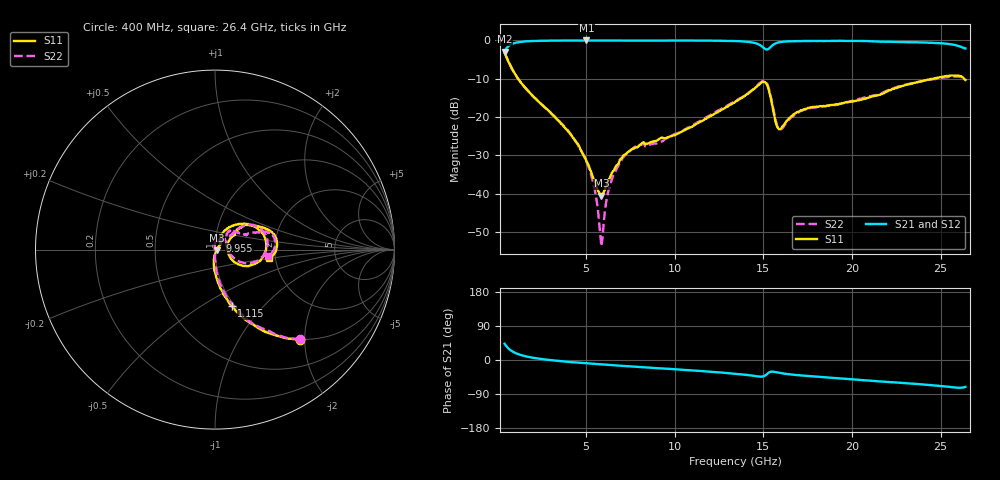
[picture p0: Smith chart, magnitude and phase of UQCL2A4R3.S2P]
! AVX Corporation
! Date:  10/27/06
! Part No:  UQCL2A4R3
! Description:  Ultra Low ESR Microwave capacitors
! Mounting Orientation:  Horizontal
# GHZ S DB R 50
! Freq  |S11|  S11 Ph  |S21|  S21 Ph  |S12|  S12 Ph  |S22|  S22 Ph
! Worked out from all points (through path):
!   401 points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, 400 MHz to 26.4 GHz, reference 50 ohm
!   highest |S21| = -0.04 dB at 5.015 GHz (marker M1); lowest = -2.9 dB at 400 MHz (marker M2)
!   group delay of S21, straight-line fit = 8.74 ps
!   lowest |S11| = -40.5 dB at 5.86 GHz (marker M3), VSWR 1.02, Z = 50.9 - j0.397 ohm
!   |S11| at or under -10 dB: 1.158 GHz to 24.58 GHz (23.42 GHz wide, 182 % of centre); 26.32633 GHz to end of sweep
!   |S22| runs from -53.7 to -3.2 dB; largest |S21 - S12| = 0.0084
!   S11 on the Smith chart (normalised r, x): 400 MHz: 0.99, -1.89; 1.115 GHz: 0.97, -0.68; 9.955 GHz: 1.05, +0.11; 26.4 GHz: 1.84, -0.20
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0.4  -3.23 -46.7  -2.93 42.7  -2.97 42.7  -3.23 -46.5
1.115  -9.72 -73.4  -0.54 16.4  -0.57 16.3  -9.69 -72.4
3.91  -23.34 -95.5  -0.06 -4.6  -0.04 -4.6  -23.16 -88.2
4.755  -29.09 -95.0  -0.05 -7.8  -0.04 -7.9  -29.14 -89.2
5.015  -31.53 -90.7  -0.04 -8.8  -0.03 -8.8  -31.63 -90.0
5.47  -36.68 -72.0  -0.04 -10.4  -0.03 -10.4  -38.60 -95.9
5.86  -40.54 -24.5  -0.04 -11.7  -0.04 -11.7  -53.72 -175.2
6.315  -36.07 23.3  -0.06 -13.2  -0.05 -13.1  -38.18 97.6
7.03  -30.59 40.2  -0.06 -15.4  -0.03 -15.5  -30.96 94.5
7.81  -27.96 44.7  -0.06 -17.8  -0.04 -18.0  -27.74 85.9
9.11  -25.76 56.9  -0.08 -21.8  -0.08 -22.0  -26.60 71.2
9.955  -24.77 61.1  -0.07 -24.3  -0.05 -24.4  -24.55 57.6
13.4  -16.13 55.5  -0.21 -36.1  -0.21 -36.1  -15.86 41.9
14.57  -12.27 33.8  -0.77 -42.7  -0.79 -42.5  -12.18 34.1
15.09  -10.92 0.2  -2.22 -41.2  -2.24 -41.2  -10.62 5.1
15.415  -14.98 -30.5  -1.73 -31.1  -1.75 -31.1  -14.55 -23.9
15.74  -22.09 -18.4  -0.71 -32.4  -0.73 -32.3  -21.78 -12.4
15.935  -23.20 7.0  -0.48 -34.2  -0.49 -34.1  -23.42 14.0
17.755  -17.43 37.0  -0.17 -43.2  -0.16 -43.1  -17.63 52.0
22.11  -13.00 38.4  -0.38 -58.2  -0.37 -58.2  -12.88 24.6
25.23  -9.41 14.9  -0.86 -69.6  -0.85 -69.3  -9.70 15.9
26.4  -10.36 -9.3  -2.12 -71.0  -2.10 -71.3  -10.45 -7.1
